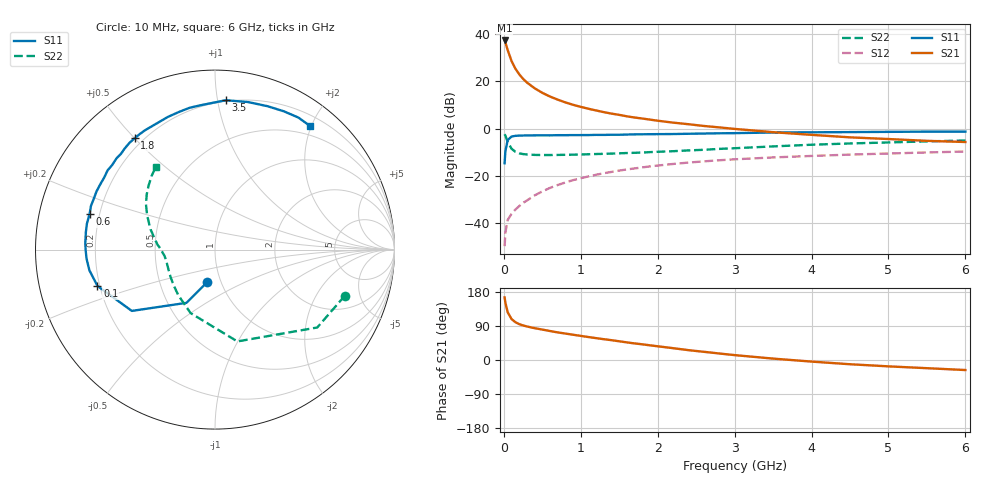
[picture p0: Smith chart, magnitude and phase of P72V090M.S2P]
! SIEMENS Small Signal Semiconductors
! BFP196
! Si NPN RF Bipolar Junction Transistor in SOT143
! VCE = 2 V  IC = 90 mA
! Common Emitter S-Parameters:  May  1996
# GHz  S  MA  R  50
!  f  S11  S21  S12  S22
! GHz  MAG  ANG  MAG  ANG  MAG  ANG  MAG  ANG
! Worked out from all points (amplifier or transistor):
!   36 points, 10 MHz to 6 GHz, reference 50 ohm
!   highest |S21| = 37.3 dB at 10 MHz (marker M1)
!   |S21| within 3 dB of that: start of sweep to 40.19 MHz
!   unconditionally stable (mu >= 1): 277.4 MHz to 5.26 GHz; 5.789 GHz to end of sweep
!   at 250 MHz: K = 0.97, MSG = 26.2 dB, |S12| = -31.3 dB
!   at 1.4 GHz: K = 1.11, MAG = 10.3 dB, |S12| = -18.2 dB
!   at 6 GHz: K = 1.00, MAG = 1.7 dB, |S12| = -9.6 dB
!   S11 on the Smith chart (normalised r, x): 10 MHz: 0.86, -0.32; 100 MHz: 0.19, -0.15; 600 MHz: 0.16, +0.14; 1.8 GHz: 0.17, +0.50; 3.5 GHz: 0.19, +1.06; 6 GHz: 0.35, +1.99
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0.01  0.1871 -103.6  73.61 165.2  0.0033 73.4  0.7675 -19.6
0.02  0.3366 -118.2  66.99 151.4  0.0064 65.6  0.7161 -37.3
0.05  0.5757 -143.6  46.13 126.0  0.0118 53.3  0.5266 -76.3
0.1  0.6853 -162.8  27.05 108.0  0.0159 51.6  0.379 -111.0
0.15  0.7092 -170.6  18.67 99.8  0.0196 55.4  0.3263 -128.8
0.2  0.7173 -175.9  14.2 94.6  0.0232 59.0  0.3033 -139.7
0.25  0.7207 -179.7  11.36 91.2  0.0272 60.9  0.2917 -147.5
0.3  0.7237 177.1  9.517 88.5  0.0305 63.6  0.2863 -152.3
0.4  0.7261 172.1  7.188 84.0  0.0391 65.6  0.2804 -159.3
0.5  0.7281 168.6  5.756 80.3  0.0474 66.6  0.2788 -163.8
0.6  0.7263 164.2  4.801 76.5  0.0563 66.8  0.2789 -166.8
0.7  0.7328 160.5  4.131 72.8  0.0647 66.3  0.2801 -169.1
0.8  0.7324 157.1  3.609 69.8  0.0733 65.3  0.2817 -171.0
1.1  0.7364 147.0  2.65 60.6  0.0983 62.5  0.2894 -175.4
1.4  0.748 137.2  2.092 52.3  0.1225 58.0  0.2987 -179.0
1.8  0.765 125.7  1.647 41.4  0.1527 51.8  0.3143 176.5
2.2  0.7741 115.0  1.349 31.2  0.1804 45.5  0.3356 171.3
2.8  0.8029 100.0  1.07 17.2  0.2159 36.2  0.3755 162.7
3.5  0.8343 85.9  0.847 3.7  0.248 26.0  0.4241 153.1
4.5  0.8509 69.9  0.659 -11.2  0.2845 13.7  0.4894 141.0
5.5  0.8701 57.7  0.556 -21.6  0.3159 2.9  0.5412 130.8
6  0.8689 52.3  0.525 -26.5  0.3305 -2.8  0.5652 125.8
